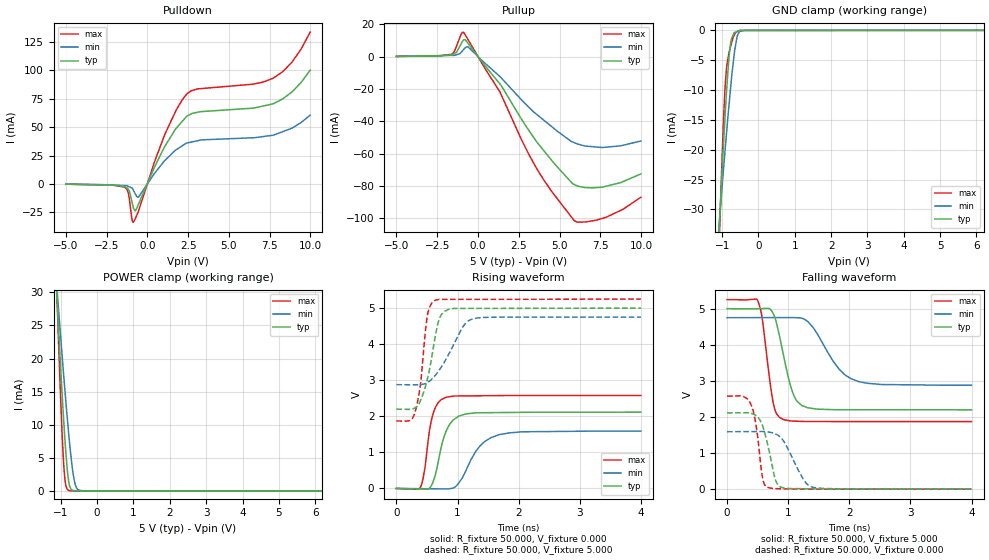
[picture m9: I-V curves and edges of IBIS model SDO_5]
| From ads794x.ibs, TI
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|   SDO 5V Model
[Model] SDO_5
Model_type   3-state
Polarity   Non-Inverting
Enable   Active-Low
Vmeas = 2.5
Vref = 2.5
Cref = 15pF
Rref = 50
|   typ   min   max
|   (Nom PVT)   (Fast PVT)  (Slow PVT)
|   (high input impedance)
C_comp   1.4494500e-12   1.1868900e-12   1.7240750e-12
|   (high output)
|C_comp   1.8572750e-12   1.6032320e-12   2.1290470e-12
|   (low output)
|C_comp   9.4931990e-13   8.5043930e-13   1.1852390e-12
[Voltage Range]   5   4.75   5.25
[Temperature Range]   27   125   -40
[Pullup Reference]   5   4.75   5.25
[Pulldown Reference]   0   0   0
[Power Clamp Reference]   5   4.75   5.25
[GND Clamp Reference]   0   0   0
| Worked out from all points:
|   slope of the pulldown table from 0 to 0.75 V, typ, clamps not added: 31.7 ohm
|   slope of the pullup table from 0 to 0.75 V, typ, clamps not added: 77.8 ohm
|   GND clamp passes 1 mA (typ) near -0.71 V on its own axis
|   POWER clamp passes 1 mA (typ) near -0.77 V on its own axis
|   falling waveform, R_fixture 50.000, V_fixture 5.000: 20-80 % time 227ps typ, 428ps min, 152ps max; typ from 5 V to 2.2 V
|   rising waveform, R_fixture 50.000, V_fixture 0.000: 20-80 % time 200ps typ, 341ps min, 137ps max; typ from 0 V to 2.11 V
|   rising waveform, R_fixture 50.000, V_fixture 5.000: 20-80 % time 199ps typ, 365ps min, 127ps max; typ from 2.2 V to 5 V
|   falling waveform, R_fixture 50.000, V_fixture 0.000: 20-80 % time 172ps typ, 286ps min, 119ps max; typ from 2.11 V to 0 V
[Pulldown]
|   Voltage   I(typ)   I(min)   I(max)
-5V       -245.1uA   -183.6uA   -242.9uA
-1.396V   -2.339mA   -1.389mA   -2.808mA
-1.169V   -4.818mA   -2.106mA   -7.752mA
-950.8mV  -15.28mA   -3.538mA   -30.48mA
-861.8mV  -20.61mA   -5.33mA    -33.73mA
-744.9mV  -23.75mA   -8.539mA   -30.82mA
-534.2mV  -17.57mA   -11.44mA   -23.61mA
1.079V    33.25mA    20.73mA    43.91mA
2.404V    59.43mA    36.01mA    79.08mA
7.651V    70.42mA    42.79mA    92.77mA
8.845V    80.85mA    49.01mA    107mA
9.985V    100.3mA    60.66mA    133.8mA
[GND Clamp]
|   Voltage   I(typ)   I(min)   I(max)
-5V       -577.7mA   -377.4mA   -895.1mA
-1.085V   -33.68mA   -32.82mA   -36.88mA
-1.055V   -30.15mA   -30.53mA   -31.18mA
-950.8mV  -18mA      -22.49mA   -13.64mA
-907.9mV  -13.34mA   -19.38mA   -8.593mA
-874.2mV  -9.924mA   -16.95mA   -6.164mA
-811.7mV  -4.639mA   -12.65mA   -3.831mA
-744.9mV  -1.493mA   -8.268mA   -2.228mA
-655mV    -352.7uA   -3.392mA   -671.8uA
-592.1mV  -210uA     -1.201mA   -241.6uA
-519.7mV  -45.61uA   -244.7uA   -23.43uA
9.985V    0A         0A         0A
[Pullup]
|   Voltage   I(typ)   I(min)   I(max)
-5V       134uA      109uA      143uA
-1.661V   1.047mA    749.4uA    1.343mA
-1.324V   2.585mA    1.146mA    6.274mA
-907.9mV  9.969mA    4.098mA    15.18mA
-579.1mV  7.825mA    5.719mA    9.997mA
1.341V    -16.84mA   -12.28mA   -21.78mA
2.669V    -38.71mA   -26.77mA   -51.46mA
3.607V    -52.86mA   -35.82mA   -69.41mA
5.909V    -79.13mA   -53.27mA   -101.6mA
6.552V    -81.03mA   -55.28mA   -102.3mA
7.837V    -80.22mA   -56.04mA   -99.42mA
9.985V    -72.57mA   -52.19mA   -86.99mA
[POWER Clamp]
|   Voltage   I(typ)   I(min)   I(max)
-5V       504.4mA    359.8mA    727.2mA
-1.114V   30.26mA    31.25mA    30.83mA
-1.082V   26.88mA    28.9mA     25.69mA
-992.7mV  17.52mA    22.5mA     12.35mA
-922.5mV  10.84mA    17.59mA    4.258mA
-867.8mV  6.315mA    13.98mA    1.056mA
-777.4mV  1.265mA    8.369mA    57.56uA
-681.6mV  115.5uA    3.393mA    4.567uA
-612.1mV  12.07uA    1.172mA    4.538uA
-534.2mV  3.587uA    195.8uA    4.504uA
-399.7mV  3.541uA    4.302uA    4.447uA
9.985V    0A         0A         0A
[Ramp]
R_load = 50
|   typ   min   max
dV/dt_r   1.26823/1.97293e-010  0.954425/3.37351e-010   1.5462/1.36764e-010
dV/dt_f   1.77214/2.25429e-010   1.13838/4.2326e-010   2.0803/1.51054e-010
[Falling Waveform]
R_fixture = 50.000
V_fixture = 5.000
V_fixture_min = 4.750
V_fixture_max = 5.250
C_fixture = 0.000
|  time   V(typ)   V(min)   V(max)
0s        4.998V     4.748V     5.249V
500.9ps   4.996V     4.75V      5.223V
573.6ps   5.001V     4.75V      4.754V
759.7ps   4.844V     4.751V     2.355V
930.6ps   3.651V     4.751V     1.923V
1.105ns   2.549V     4.75V      1.884V
1.323ns   2.253V     4.639V     1.874V
1.746ns   2.201V     3.519V     1.872V
2.024ns   2.2V       3.062V     1.871V
4ns       2.197V     2.877V     1.871V
[Rising Waveform]
R_fixture = 50.000
V_fixture = 0.000
V_fixture_min = 0.000
V_fixture_max = 0.000
C_fixture = 0.000
|  time   V(typ)   V(min)   V(max)
0s        1.791uV    -1.13uV    -337.7nV
390ps     -12.34mV   -5.979mV   22.71mV
454.9ps   -14.39mV   -6.973mV   447mV
544.3ps   12.88mV    -8.344mV   1.633V
597.3ps   172.5mV    -9.155mV   2.054V
813.6ps   1.589V     -12.47mV   2.528V
1.024ns   2.006V     161.8mV    2.563V
1.366ns   2.098V     1.176V     2.569V
1.678ns   2.103V     1.489V     2.574V
4ns       2.114V     1.591V     2.577V
[Rising Waveform]
R_fixture = 50.000
V_fixture = 5.000
V_fixture_min = 4.750
V_fixture_max = 5.250
C_fixture = 0.000
|  time   V(typ)   V(min)   V(max)
0s        2.197V     2.877V     1.871V
296.9ps   2.228V     2.874V     2.071V
392.5ps   2.431V     2.874V     2.878V
505.7ps   3.027V     2.938V     4.779V
632.2ps   4.179V     3.128V     5.216V
700.3ps   4.694V     3.282V     5.241V
784.3ps   4.904V     3.499V     5.241V
1.088ns   4.99V      4.479V     5.241V
1.233ns   4.991V     4.69V      5.241V
4ns       4.998V     4.748V     5.249V
[Falling Waveform]
R_fixture = 50.000
V_fixture = 0.000
V_fixture_min = 0.000
V_fixture_max = 0.000
C_fixture = 0.000
|  time   V(typ)   V(min)   V(max)
0s        2.114V     1.591V     2.577V
384.8ps   2.105V     1.595V     2.37V
480.9ps   2.029V     1.596V     1.697V
576.7ps   1.777V     1.597V     352.2mV
644.8ps   1.375V     1.593V     63.24mV
787.1ps   283.4mV    1.53V      15.78mV
924.9ps   33.16mV    1.332V     8.308mV
1.247ns   12.95mV    276.4mV    2.113mV
1.388ns   10.45mV    59mV       1.429mV
4ns       1.791uV    -1.13uV    -337.7nV
